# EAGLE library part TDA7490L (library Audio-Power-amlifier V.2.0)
The TDA7490L is a dual audio class D amplifier assembled in Flexiwatt 25 package; it is specially designed for high efficiency application mainly for TV and Home Stereo sets.
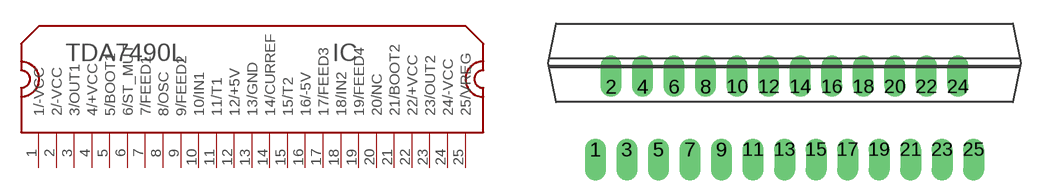
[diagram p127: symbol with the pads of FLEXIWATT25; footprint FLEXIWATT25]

Designator prefix IC

## TDA7490L  [FLEXIWATT25]
1  1/-VCC  pwr
2  2/-VCC  pwr
3  3/OUT1  out
4  4/+VCC  pwr
5  5/BOOT1
6  6/ST_MUT
7  7/FEED1
8  8/OSC
9  9/FEED2
10  10/IN1  in
11  11/T1
12  12/+5V  pwr
13  13/GND  pwr
14  14/CURREF
15  15/T2
16  16/-5V  pwr
17  17/FEED3
18  18/IN2  in
19  19/FEED4
20  20/NC  nc
21  21/BOOT2
22  22/+VCC  pwr
23  23/OUT2  out
24  24/-VCC  pwr
25  25/VREG

## Footprint FLEXIWATT25 (pad centres in mm)
Flexiwatt25 (vertical)
drill 0.813 offset: 1 -12,0; 2 -11,4; 3 -10,0; 4 -9,4; 5 -8,0; 6 -7,4; 7 -6,0; 8 -5,4; 9 -4,0; 10 -3,4; 11 -2,0; 12 -1,4; 13 0,0; 14 1,4; 15 2,0; 16 3,4; 17 4,0; 18 5,4; 19 6,0; 20 7,4; 21 8,0; 22 9,4; 23 10,0; 24 11,4; 25 12,0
